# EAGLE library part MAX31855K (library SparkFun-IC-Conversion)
Cold-Junction-Compensated K-Thermocoupleto-Digital Converter (-270°C to +1800°C) The MAX31855K performs cold-junction compensation and digitizes the signal from a type-K thermocouple. The data is output in a 14-bit resolution, SPI™-compatible, read-only format. This converter resolves temperatures to 0.25°C, allows readings as high as +1800°C and as low as -270°C, and exhibits thermocouple accuracy of ±2°C for temperatures ranging from -200°C to +700°C for K-type thermocouples. Datasheet SparkFun Products SparkFun Thermocouple Breakout - MAX31855K (SEN-13266)
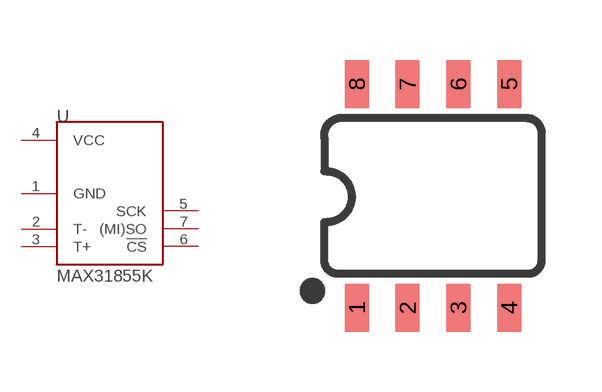
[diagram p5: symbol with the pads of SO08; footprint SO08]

Designator prefix U

## MAX31855K (PROD_ID: IC-12578; VALUE: MAX31855K)  [SO08]
1  GND
2  T-
3  T+
4  VCC
5  SCK
6  !CS
7  (MI)SO

## Footprint SO08 (pad centres in mm)
SOIC, 0.15 inch width
smd 0.6 x 1.2: 1 -1.905,-2.8; 2 -0.635,-2.8; 3 0.635,-2.8; 4 1.905,-2.8; 5 1.905,2.8; 6 0.635,2.8; 7 -0.635,2.8; 8 -1.905,2.8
